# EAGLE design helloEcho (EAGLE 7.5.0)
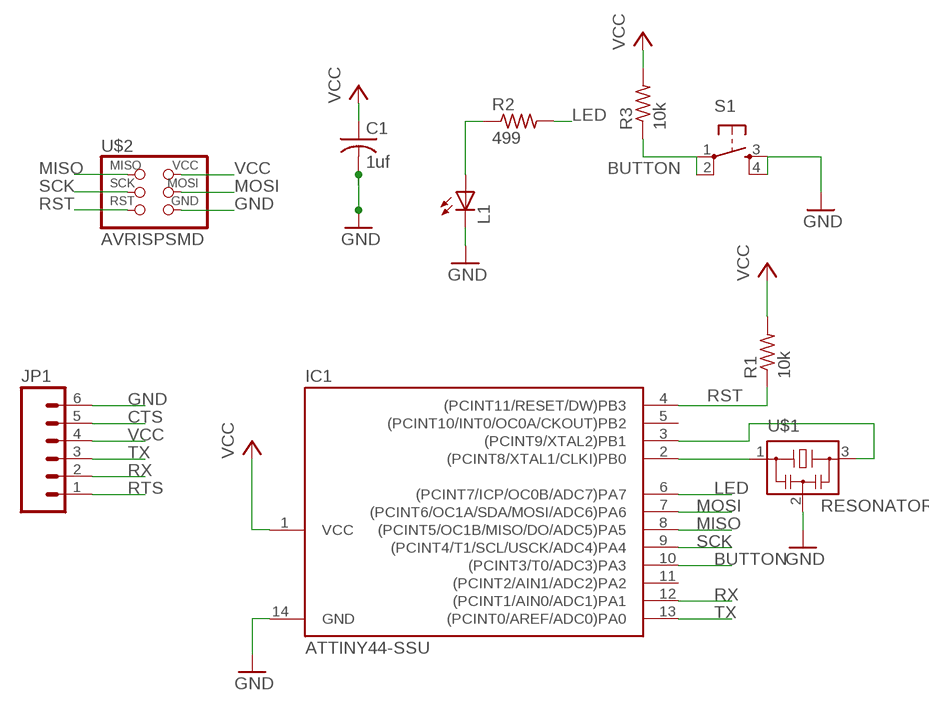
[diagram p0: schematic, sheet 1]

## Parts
C1  1uf  C-USC1206  [C1206]
IC1  ATTINY44-SSU  [SOIC14]
JP1  M06SMD  [1X06-SMD]
L1  LED1206  [1206]
R1  10k  R-US_R1206  [R1206]
R2  499  RESISTOR1206  [1206]
R3  10k  R-US_R1206  [R1206]
S1  6MM_SWITCH6MM_SWITCH  [6MM_SWITCH]
U$1  RESONATOR  [EFOBM]
U$2  AVRISPSMD  [2X03SMD]

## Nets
BUTTON: IC1.10((PCINT3/T0/ADC3)PA3) R3.1 S1.1(P) S1.2(P1)
CTS: JP1.5
GND: C1.2 IC1.14(GND) JP1.6 L1.2(C) S1.3(S) S1.4(S1) U$1.2 U$2.6(GND)
LED: IC1.6((PCINT7/ICP/OC0B/ADC7)PA7) R2.2
MISO: IC1.8((PCINT5/OC1B/MISO/DO/ADC5)PA5) U$2.1(MISO)
MOSI: IC1.7((PCINT6/OC1A/SDA/MOSI/ADC6)PA6) U$2.4(MOSI)
N$1: IC1.2((PCINT8/XTAL1/CLKI)PB0) U$1.1
N$2: IC1.3((PCINT9/XTAL2)PB1) U$1.3
N$4: L1.1(A) R2.1
RST: IC1.4((PCINT11/RESET/DW)PB3) R1.1 U$2.5(RST)
RTS: JP1.1
RX: IC1.12((PCINT1/AIN0/ADC1)PA1) JP1.2
SCK: IC1.9((PCINT4/T1/SCL/USCK/ADC4)PA4) U$2.3(SCK)
TX: IC1.13((PCINT0/AREF/ADC0)PA0) JP1.3
VCC: C1.1 IC1.1(VCC) JP1.4 R1.2 R3.2 U$2.2(VCC)
Unconnected: IC1.5((PCINT10/INT0/OC0A/CKOUT)PB2) IC1.11((PCINT2/AIN1/ADC2)PA2)

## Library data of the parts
C1 = rcl:C-US: CAPACITOR, American symbol
IC1 = fab:ATTINY44
JP1 = SparkFun:M06: Header 6 Standard 6-pin 0.1" header. Use with straight break away headers (SKU : PRT-00116), right angle break away headers (PRT-00553), swiss pins (PRT-00743), machine pins (PRT-00117), and female headers (PRT-00115). Molex polarized connector foot print use with SKU : PRT-08094 with associated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
L1 = 01_FAB_Hello:LED
R1 R3 = resistor:R-US_: RESISTOR, American symbol
R2 = 01_FAB_Hello:RESISTOR
S1 = 01_FAB_Hello:6MM_SWITCH: OMRON SWITCH
U$1 = fab:RESONATOR
U$2 = fab:AVRISP

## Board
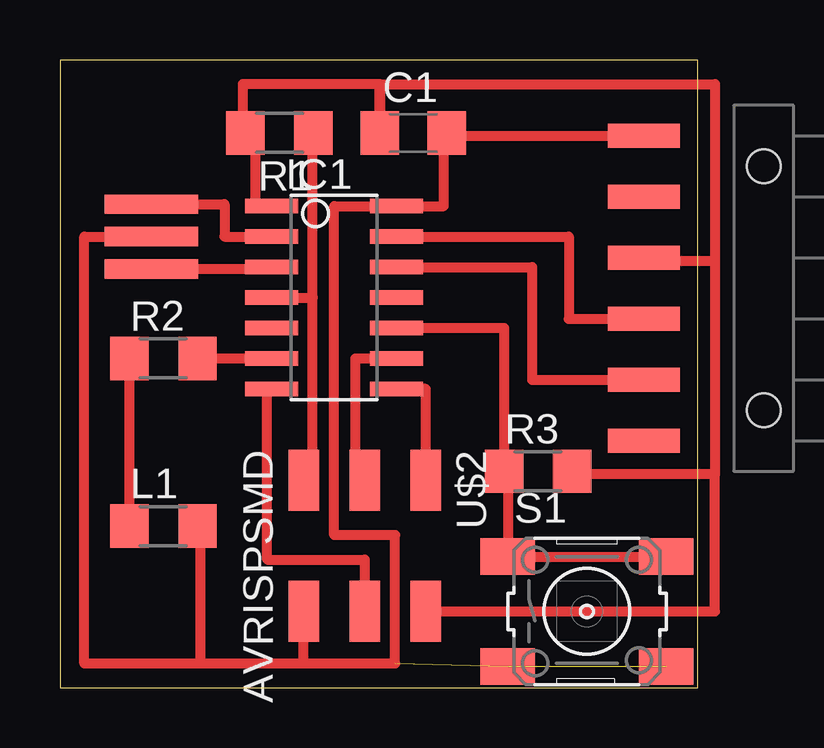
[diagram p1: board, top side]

Size 26.59 x 26.15 mm. Coordinates in mm from the lower left corner, seen from the top.
Outline: 0,0 26.59,0 26.59,26.15 0,26.15 0,0
Copper layers 1: Top 0.035mm
Design rules "ERP-1sided-10mil-16mill": minimum track width 10mil, minimum drill 24mil, track to track 16mil, track to pad 16mil, pad to pad 16mil, via to via 16mil, smd to smd 0mil, copper to edge 16mil, drill to drill 36mil, minimum pad ring 10mil, minimum via ring 8mil, stop-mask expansion 4mil, vias tented up to drill 0mil, thermal gap 10mil

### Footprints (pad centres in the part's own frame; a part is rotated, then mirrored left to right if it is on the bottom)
C1206 = smd 1.6 x 1.8: 1 -1.4,0; 2 1.4,0
SOIC14 = smd 0.61 x 2.21: 1 -3.81,-2.603; 2 -2.54,-2.603; 3 -1.27,-2.603; 4 0,-2.603; 5 1.27,-2.603; 6 2.54,-2.603; 7 3.81,-2.603; 8 3.81,2.603; 9 2.54,2.603; 10 1.27,2.603; 11 0,2.603; 12 -1.27,2.603; 13 -2.54,2.603; 14 -3.81,2.603
1X06-SMD = smd 1 x 3: 1 -6.35,5; 2 -3.81,5; 3 -1.27,5; 4 1.27,5; 5 3.81,5; 6 6.35,5 | hole 1.4: -5.08,0; 5.08,0
1206 = smd 1.6 x 1.803: 1 -1.422,0; 2 1.422,0
R1206 = smd 1.6 x 1.803: 1 -1.422,0; 2 1.422,0
6MM_SWITCH = smd 2.286 x 1.524: 1 -3.302,2.286; 2 3.302,2.286; 3 -3.302,-2.286; 4 3.302,-2.286
EFOBM = smd 0.8 x 3.9: 1 -1.35,0; 2 0,0; 3 1.35,0
2X03SMD = smd 2.54 x 1.27: 1 -2.54,2.54; 2 2.92,2.54; 3 -2.54,0; 4 2.92,0; 5 -2.54,-2.54; 6 2.92,-2.54

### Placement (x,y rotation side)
C1  14.73,23.11 0 top
IC1  11.43,16.26 270 top
JP1  29.34,16.64 90 top
L1  4.32,6.73 0 top
R1  9.14,23.11 180 top
R2  4.32,13.72 0 top
R3  19.94,9.02 0 top
S1  21.97,3.17 0 top
U$1  3.81,18.8 270 top
U$2  12.7,6.1 270 top

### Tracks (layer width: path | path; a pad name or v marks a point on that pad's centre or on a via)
BUTTON
  Top 0.406: S1.2 S1.1 18.67,9.02 R3.1 18.52,14.99 IC1.10
GND  (2 unrouted)
  Top 0.406: 10.16,1.02 13.97,1.02 13.97,6.35 11.43,6.35 11.43,20.07 IC1.14 16,20.07 16,23.11 C1.2 16.13,22.99 JP1.6 | U$1.2 1.02,18.8 1.02,1.02 5.84,1.02 | U$2.6 10.16,1.02 | 5.84,1.02 10.16,1.02 | L1.2 5.84,6.73 5.84,1.02
LED
  Top 0.406: R2.2 IC1.6
MISO
  Top 0.406: IC1.8 15.24,12.45 U$2.1
MOSI
  Top 0.406: IC1.7 8.64,12.45 8.64,5.33 12.7,5.33 U$2.4
N$1
  Top 0.406: U$1.1 6.86,20.15 6.86,18.8 IC1.2
N$2
  Top 0.406: U$1.3 8.83,17.45 IC1.3
N$4
  Top 0.406: L1.1 R2.1
RST
  Top 0.406: R1.1 10.54,23.11 10.54,16.26 | IC1.4 10.54,16.26 | U$2.5 10.54,8.64 10.54,16.26
RX
  Top 0.406: IC1.12 19.68,17.53 19.68,12.83 JP1.2
SCK
  Top 0.406: U$2.3 12.32,8.64 12.32,13.72 IC1.9
TX
  Top 0.406: IC1.13 21.21,18.8 21.21,15.37 JP1.3
VCC
  Top 0.406: IC1.1 8.13,20.07 8.13,23.11 R1.2 7.62,23.11 7.62,25.15 13.33,25.15 C1.1 13.34,25.15 27.3,25.15 27.3,17.78 | JP1.4 24.34,17.78 27.3,17.78 | 27.3,17.78 27.3,8.89 | 27.3,8.89 21.36,8.89 R3.2 | U$2.2 27.3,3.18 27.3,8.89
